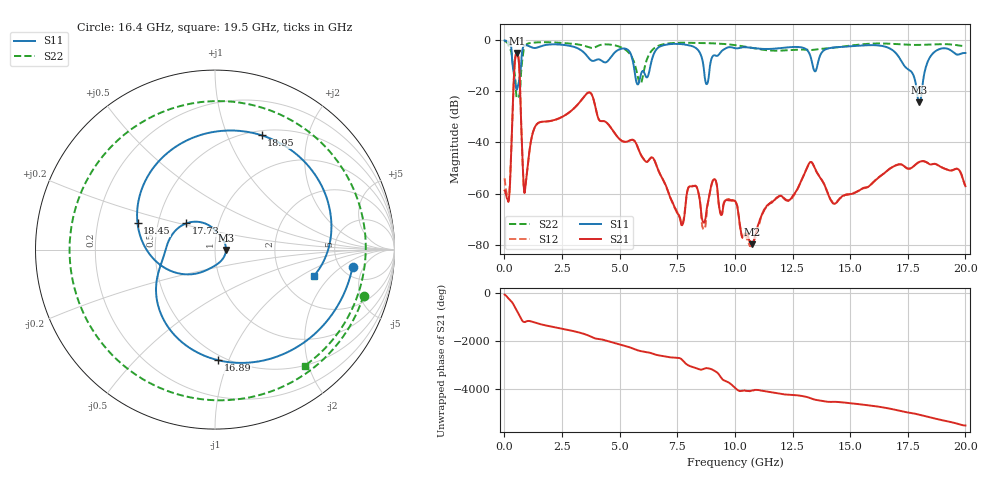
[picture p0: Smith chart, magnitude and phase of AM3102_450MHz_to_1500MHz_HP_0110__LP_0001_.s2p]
!Agilent Technologies,E8364B,MY43040894,A.07.50.67
!Agilent E8364B: A.07.50.67
!Date: Thursday, January 11, 2018 05:44:51
!Correction: S11(Full 2 Port(1,2))
!S21(Full 2 Port(1,2))
!S12(Full 2 Port(1,2))
!S22(Full 2 Port(1,2))
!S2P File: Measurements: S11, S21, S12, S22:
# Hz S  dB  R 50
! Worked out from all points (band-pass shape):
!   1601 points, 10 MHz to 20 GHz, reference 50 ohm
!   highest |S21| = -4.93 dB at 534.7 MHz (marker M1); lowest = -79.8 dB at 10.74 GHz (marker M2)
!   |S21| within 3 dB of the highest: 459.5 MHz to 624.4 MHz (164.9 MHz wide, 30.4 % of centre)
!   lowest |S11| = -24.3 dB at 18 GHz (marker M3), VSWR 1.13, Z = 56.5 - j0.265 ohm
!   |S11| at or under -10 dB: 361.9 MHz to 721.7 MHz (359.8 MHz wide, 66.4 % of centre); 5.611 GHz to 6.337 GHz (725.5 MHz wide, 12.1 % of centre); 17.35 GHz to 18.3 GHz (949.1 MHz wide, 5.32 % of centre)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
!   |S22| runs from -22.5 to -0.3 dB; largest |S21 - S12| = 0.0015
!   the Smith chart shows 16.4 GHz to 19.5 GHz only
!   S11 on the Smith chart (normalised r, x): 16.4 GHz: 6.27, -3.05; 16.89 GHz: 0.46, -0.91; 17.73 GHz: 0.70, +0.21; 18.45 GHz: 0.38, +0.14; 18.95 GHz: 0.55, +1.34; 19.5 GHz: 3.03, -1.31
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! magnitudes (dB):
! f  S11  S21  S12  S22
! 10 MHz  -0.1  -58.8  -54.0  -0.3
! 209.9 MHz  -0.8  -61.0  -60.6  -2.8
! 534.7 MHz  -19.4  -4.9  -4.9  -22.4
! 897.1 MHz  -1.9  -58.5  -58.2  -2.1
! 1.384 GHz  -2.9  -33.1  -33.1  -0.8
! 3.346 GHz  -4.0  -23.4  -23.4  -1.9
! 5.895 GHz  -14.3  -44.3  -44.4  -17.0
! 6.682 GHz  -2.8  -51.0  -50.9  -2.2
! 7.694 GHz  -1.5  -72.3  -72.1  -1.0
! 10.01 GHz  -3.1  -62.9  -63.1  -1.9
! 10.74 GHz  -3.0  -79.8  -80.0  -3.0
! 13.34 GHz  -8.4  -47.9  -47.9  -3.8
! 14.3 GHz  -2.8  -64.1  -63.6  -2.9
! 16.4 GHz  -2.2  -52.6  -52.6  -1.2
! 16.68 GHz  -3.0  -50.5  -50.6  -1.3
! 16.89 GHz  -4.2  -49.4  -49.2  -1.4
! 17.73 GHz  -13.3  -49.5  -49.6  -1.8
! 18 GHz  -24.3  -47.6  -47.6  -1.8
! 18.45 GHz  -6.8  -48.5  -48.4  -1.7
! 18.95 GHz  -3.2  -49.7  -49.7  -1.5
! 19.5 GHz  -4.9  -50.7  -50.6  -1.7
! 20 GHz  -5.0  -57.1  -56.9  -2.3
